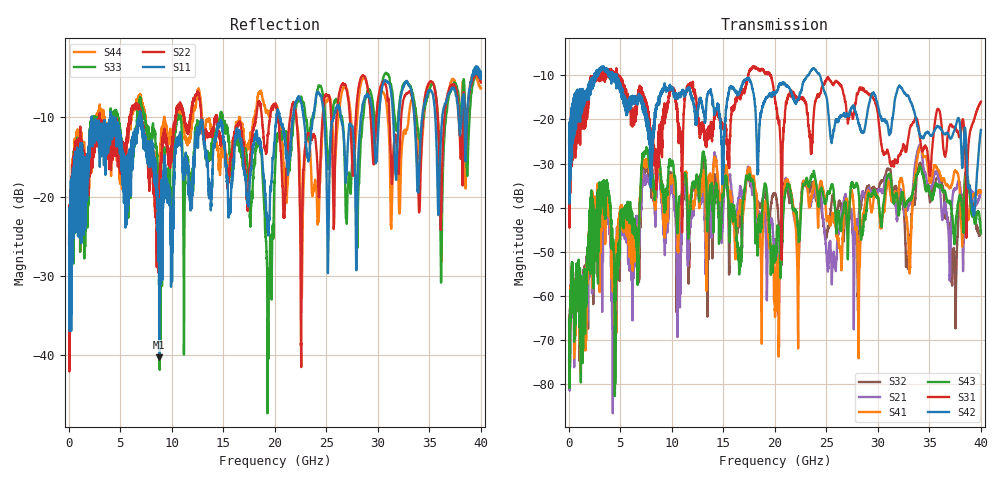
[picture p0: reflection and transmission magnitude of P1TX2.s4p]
!Agilent Technologies,N5245A,MY49151084,A.09.20.08
!Agilent N5245A: A.09.20.08
!Date: Thursday, March 01, 2012 14:02:30
!Correction: S11(Full 4 Port(1,2,3,4))
!S12(Full 4 Port(1,2,3,4))
!S13(Full 4 Port(1,2,3,4))
!S14(Full 4 Port(1,2,3,4))
!S21(Full 4 Port(1,2,3,4))
!S22(Full 4 Port(1,2,3,4))
!S23(Full 4 Port(1,2,3,4))
!S24(Full 4 Port(1,2,3,4))
!S31(Full 4 Port(1,2,3,4))
!S32(Full 4 Port(1,2,3,4))
!S33(Full 4 Port(1,2,3,4))
!S34(Full 4 Port(1,2,3,4))
!S41(Full 4 Port(1,2,3,4))
!S42(Full 4 Port(1,2,3,4))
!S43(Full 4 Port(1,2,3,4))
!S44(Full 4 Port(1,2,3,4))
!S4P File: Measurements: <S11,S12,S13,S14>,
!<S21,S22,S23,S24>,
!<S31,S32,S33,S34>,
!<S41,S42,S43,S44>:
# Hz S  dB  R 50
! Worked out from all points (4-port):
!   3996 points, 50 MHz to 40 GHz, reference 50 ohm
!   strongest paths, dB at 50 MHz, 10.04 GHz, 20.03 GHz, 30.02 GHz, 40 GHz:
!     S42: -25.0, -12.9, -14.2, -16.9, -22.4
!     S31: -25.6, -13.0, -15.5, -18.9, -16.0
!     S43: -65.1, -29.5, -51.0, -37.6, -45.8
!     S41: -70.4, -33.2, -64.7, -37.9, -36.3
!     S21: -74.9, -34.9, -48.1, -36.1, -36.5
!     S32: -74.4, -32.3, -37.0, -36.0, -45.2
!   lowest |S11| = -40.3 dB at 8.79 GHz (marker M1), VSWR 1.02, Z = 49.4 - j0.741 ohm
!   |S11| at or under -10 dB: start of sweep to 2.237 GHz; 4.41 GHz to 6.858 GHz (2.447 GHz wide, 43.4 % of centre); 7.031 GHz to 20.14 GHz (13.11 GHz wide, 96.5 % of centre)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
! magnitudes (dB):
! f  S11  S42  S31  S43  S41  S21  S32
! 50 MHz  -23.9  -25.0  -25.6  -65.1  -70.4  -74.9  -74.4
! 2.68 GHz  -11.2  -9.8  -10.3  -42.0  -38.7  -40.5  -44.6
! 8.79 GHz  -40.3  -16.7  -21.6  -29.3  -30.4  -33.1  -31.3
! 17.57 GHz  -18.3  -11.1  -8.8  -32.7  -30.9  -32.3  -33.8
! 20.23 GHz  -9.5  -13.5  -18.5  -44.3  -52.2  -51.2  -39.4
! 21.16 GHz  -15.2  -12.4  -15.9  -35.6  -33.6  -33.8  -35.5
! 40 GHz  -5.1  -22.4  -16.0  -45.8  -36.3  -36.5  -45.2
